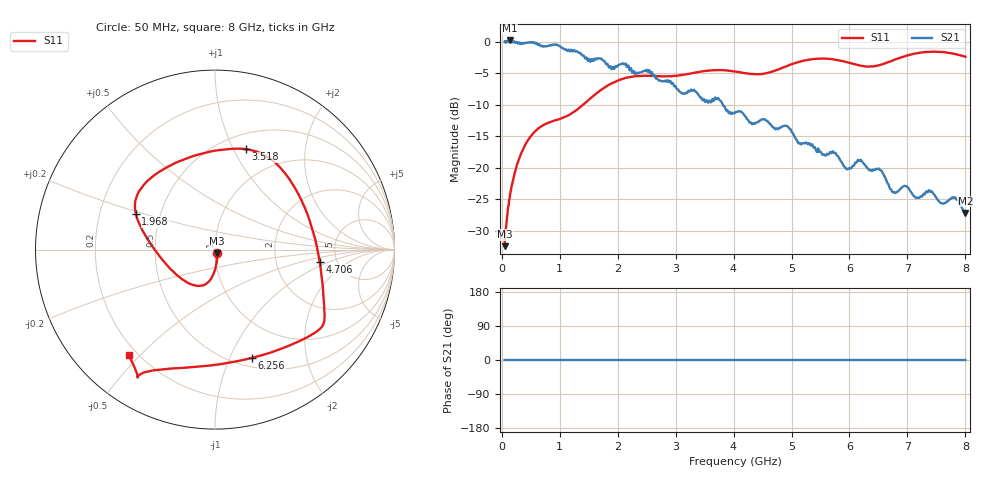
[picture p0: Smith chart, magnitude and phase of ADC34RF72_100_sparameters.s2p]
! Texas Instruments, Inc.
! ADC34RF72 - Single Channel S-Parameters - Fs = 1.5 GSPS, Termination = 100
! Port 1 represents the 100-ohm differential input, Port 2 represents the digital output of the ADC
! freq  magS11  angS11  magS21  angS21  magS12  angS12  magS22  angS22
# Hz S ma R 100
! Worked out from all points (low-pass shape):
!   1601 points, 50 MHz to 8 GHz, reference 100 ohm
!   highest |S21| = 0.19 dB at 134.5 MHz (marker M1); lowest = -27.1 dB at 8 GHz (marker M2)
!   |S21| within 3 dB of the highest: start of sweep to 1.478 GHz; 1.632 GHz to 1.732 GHz (99.39 MHz wide, 5.91 % of centre)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
!   lowest |S11| = -32.4 dB at 50 MHz (marker M3), VSWR 1.05, Z = 102 - j4.27 ohm
!   |S11| at or under -10 dB: start of sweep to 1.403 GHz
!   S12 and S22 are empty: the file has one direction only
!   S11 on the Smith chart (normalised r, x): 50 MHz: 1.02, -0.04; 1.968 GHz: 0.36, +0.19; 3.518 GHz: 0.66, +1.12; 4.706 GHz: 3.68, -0.77; 6.256 GHz: 0.60, -1.21; 8 GHz: 0.17, -0.46
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5e7  0.02394 -60.6  1 0.0  0 0.0  0 0.0
1.344688e8  0.05672 -80.0  1.022 0.0  0 0.0  0 0.0
2.835312e8  0.1119 -89.8  0.9664 0.0  0 0.0  0 0.0
4.971875e8  0.1767 -100.0  0.982 0.0  0 0.0  0 0.0
9.095938e8  0.237 -126.7  0.9444 0.0  0 0.0  0 0.0
1.376656e9  0.3087 -172.5  0.7894 0.0  0 0.0  0 0.0
1.967938e9  0.484 155.7  0.6382 0.0  0 0.0  0 0.0
2.107062e9  0.5108 150.9  0.6613 0.0  0 0.0  0 0.0
2.703312e9  0.5321 122.7  0.4948 0.0  0 0.0  0 0.0
3.518188e9  0.5862 72.8  0.3345 0.0  0 0.0  0 0.0
4.025e9  0.5802 49.5  0.2732 0.0  0 0.0  0 0.0
4.705719e9  0.5874 -6.7  0.206 0.0  0 0.0  0 0.0
4.914406e9  0.6396 -19.9  0.2141 0.0  0 0.0  0 0.0
5.351656e9  0.7254 -32.9  0.1539 0.0  0 0.0  0 0.0
5.838594e9  0.7084 -43.6  0.1153 0.0  0 0.0  0 0.0
5.967781e9  0.685 -49.6  0.09782 0.0  0 0.0  0 0.0
6.255969e9  0.6374 -71.2  0.1069 0.0  0 0.0  0 0.0
6.534219e9  0.6543 -96.5  0.09584 0.0  0 0.0  0 0.0
6.678312e9  0.69 -106.9  0.0724 0.0  0 0.0  0 0.0
7.100656e9  0.7989 -120.5  0.06038 0.0  0 0.0  0 0.0
7.806219e9  0.8006 -123.7  0.05803 0.0  0 0.0  0 0.0
8e9  0.7587 -129.3  0.04392 0.0  0 0.0  0 0.0
